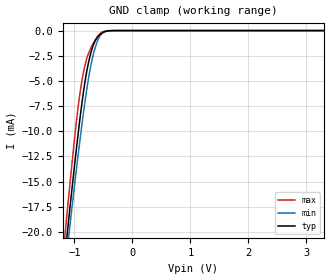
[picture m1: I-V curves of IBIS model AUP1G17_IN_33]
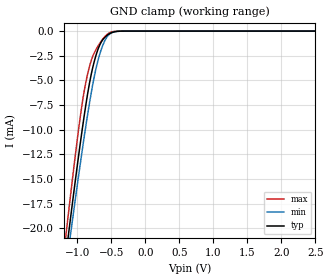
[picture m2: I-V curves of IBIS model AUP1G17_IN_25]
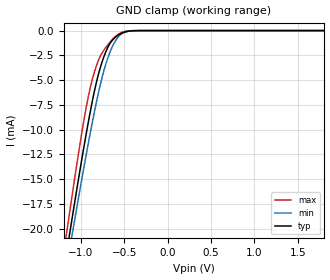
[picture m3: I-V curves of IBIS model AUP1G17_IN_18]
| TEXAS INSTRUMENTS INCORPORATED
| Standard Linear and Logic Group
| IBIS Model of SN74AUP1G17
| Low-Power Single Schmitt-Trigger Buffer
| This file contains package information for the following:
|  SOT 5-pin (DCK) package as [Component] AUP1G17_DCK
|  SOT 5-pin (DBV) package as [Component] AUP1G17_DBV
|  NanoStar WCSP 5-pin (YEP) package as [Component] AUP1G17_YEP
|  NanoFree WCSP 5-pin (YZP) package as [Component] AUP1G17_YZP
|  XSON 5-pin (DPW) package as [Component] AUP1G17_DPW
| This device can be powered at the following Vccs:
|  3.3 volt Vcc
|  2.5 volt Vcc
|  1.8 volt Vcc
|  1.5 volt Vcc
|  1.2 volt Vcc
|  0.8 volt Vcc
| This file provides unique models under the [Model Selector] for each Vcc.
| For operation at a specific Vcc, select the appropriate model after each
| [Model Selector] keyword.
[IBIS Ver]   3.2
[Comment char]  |_char
[File Name]   sn74aup1g17.ibs
[File Rev]   1.3 | a_die
[Date]   09/19/2017
[Source]   Data created from TI-SPICE simulations.
   Texas Instruments Incorporated.
   Analog-eLab, HPA
   12500 TI Blvd
   Dallas, TX -75243
   For Support e-mail: odt-pfmodeling@list.ti.com
[Notes]   The following is an IBIS list for the AUP1G17.
   - FILE REV HISTORY
   - 1.1 Release IBIS file on 04/02/04
   - 1.2 YEP and YZP packages released on 10/02/04
   - 1.3 DPW package released on 9/17/2017
   - Power clamp data deleted as there is no power-clamp diode.
   - Non-monotonic data in pullup data due to resistor at output
[Disclaimer]  This model is designed as an aid for customers of Texas Instruments
 TI and its licensors and suppliers make no warranties, either expressed
 or implied, with respect to this  model, including the warranties of
 merchantability or fitness for a particular purpose.
 The model is provided solely on an "as is" basis. The entire risk as to
 its quality and performance is with the customer.
[Copyright] (C)Copyright 2017 Texas Instruments Incorporated.
   All rights reserved.
| Component AUP1G17_DCK 5-pin SOT
[Component]   AUP1G17_DCK
[Manufacturer]   Texas Instruments, Inc.
[Package]
|   typ   min   max
R_pkg   2.000e-02   1.700e-02   2.500e-02
L_pkg   9.980e-10   8.810e-10   1.069e-09
C_pkg   1.460e-13   1.180e-13   2.050e-13
[Pin]   signal_name   model_name   R_pin   L_pin   C_pin
1   NC   NC   1.900e-02   1.069e-09   1.620e-13
2   A   AUP1G17_IN   1.800e-02   8.810e-10   1.210e-13
3   GND   GND   1.700e-02   1.031e-09   2.050e-13
4   Y   AUP1G17_OUT   2.000e-02   9.600e-10   1.240e-13
5   VCC   POWER   2.500e-02   1.049e-09   1.180e-13
| Component AUP1G17_DBV 5-pin SOT
[Component]   AUP1G17_DBV
[Manufacturer]   Texas Instruments, Inc.
[Package]
|   typ   min   max
R_pkg   2.500e-02   2.100e-02   2.900e-02
L_pkg   1.529e-09   1.312e-09   1.906e-09
C_pkg   1.560e-13   1.100e-13   2.400e-13
[Pin]   signal_name   model_name   R_pin   L_pin   C_pin
1   NC   NC   2.100e-02   1.511e-09   1.440e-13
2   A   AUP1G17_IN   2.300e-02   1.312e-09   1.380e-13
3   GND   GND   2.900e-02   1.906e-09   2.400e-13
4   Y   AUP1G17_OUT   2.600e-02   1.541e-09   1.500e-13
5   VCC   POWER   2.500e-02   1.374e-09   1.100e-13
| Component AUP1G17_YEP 5-pin NanoStar WCSP
[Component]   AUP1G17_YEP
[Manufacturer]   Texas Instruments, Inc.
[Package]
|   typ   min   max
R_pkg   0.001   0.001   0.001
L_pkg   0.021nH   0.021nH   0.021nH
C_pkg   0.046pF   0.045pF   0.047pF
[Pin]   signal_name   model_name   R_pin   L_pin   C_pin
1   DNU   NC   0.001   0.021nH   0.046pF
2   B   AUP1G17_IN   0.001   0.021nH   0.047pF
3   GND   GND   0.001   0.021nH   0.046pF
4   Y   AUP1G17_OUT   0.001   0.021nH   0.045pF
5   VCC   POWER   0.001   0.021nH   0.045pF
| Component AUP1G17_YZP 5-pin NanoStar WCSP
[Component]   AUP1G17_YZP
[Manufacturer]   Texas Instruments, Inc.
[Package]
|   typ   min   max
R_pkg   0.001   0.001   0.001
L_pkg   0.021nH   0.021nH   0.021nH
C_pkg   0.046pF   0.045pF   0.047pF
[Pin]   signal_name   model_name   R_pin   L_pin   C_pin
1   DNU   NC   0.001   0.021nH   0.046pF
2   B   AUP1G17_IN   0.001   0.021nH   0.047pF
3   GND   GND   0.001   0.021nH   0.046pF
4   Y   AUP1G17_OUT   0.001   0.021nH   0.045pF
5   VCC   POWER   0.001   0.021nH   0.045pF
| Component LVC1G38D_DPW 5-pin X2SON
[Component]   LVC1G38D_DPW
[Manufacturer]   Texas Instruments, Inc.
[Package]
|   typ   min   max
R_pkg   0.0364   0.0010   0.0518
L_pkg   0.2978n   0.0346n   0.4435n
C_pkg   0.0978p   0.0741p   0.1133p
[Pin]   signal_name   model_name   R_pin   L_pin   C_pin
1   D   LVC1G38D_IN   0.04116   0.30011n   0.10160p
2   CLK   LVC1G38D_IN   0.05181   0.44351n   0.11332p
3   GND   GND   0.00103   0.03456n   0.07412p
4   Q   LVC1G38D_OUT   0.04142   0.34311n   0.10148p
5   VCC   POWER   0.04662   0.36767n   0.09844p
| Model AUP1G17_IN
[Model Selector]   AUP1G17_IN
AUP1G17_IN_33   3.3 volt Vcc
AUP1G17_IN_25   2.5 volt Vcc
AUP1G17_IN_18   1.8 volt Vcc
AUP1G17_IN_15   1.5 volt Vcc
AUP1G17_IN_12   1.2 volt Vcc
AUP1G17_IN_08   0.8 volt Vcc
| Model AUP1G17_OUT
[Model Selector]   AUP1G17_OUT
AUP1G17_OUT_33   3.3 volt Vcc
AUP1G17_OUT_25   2.5 volt Vcc
AUP1G17_OUT_18   1.8 volt Vcc
AUP1G17_OUT_15   1.5 volt Vcc
AUP1G17_OUT_12   1.2 volt Vcc
AUP1G17_OUT_08   0.8 volt Vcc
| Models and submodels in the file (12): AUP1G17_IN_33 (Input), AUP1G17_IN_25 (Input), AUP1G17_IN_18 (Input), AUP1G17_IN_15 (Input), AUP1G17_IN_12 (Input), AUP1G17_IN_08 (Input), AUP1G17_OUT_33 (Output), AUP1G17_OUT_25 (Output), AUP1G17_OUT_18 (Output), AUP1G17_OUT_15 (Output), AUP1G17_OUT_12 (Output), AUP1G17_OUT_08 (Output)
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[Model]   AUP1G17_IN_33
Model_type  Input
Vinl=0.9
Vinh=2.1
| variable   typ   min   max
C_comp   1.44pF   1.17pF   1.80pF
[Temperature Range]   40   100   -40
| Ambient temperature   25   85   -40
[Voltage range]   3.3   3   3.6
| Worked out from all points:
|   GND clamp passes 1 mA (typ) near -0.64 V on its own axis
[GND Clamp]
| AUP1G17_IN_33
|   Voltage   I(typ)   I(min)   I(max)
-3.6V     -171.6mA   -163.5mA   -181.1mA
-1.16V    -22.22mA   -23.69mA   -20.18mA
-1.11V    -19.45mA   -21.09mA   -17.19mA
-1.085V   -18.08mA   -19.81mA   -15.71mA
-940mV    -10.5mA    -12.6mA    -7.822mA
-890mV    -8.117mA   -10.26mA   -5.698mA
-835mV    -5.768mA   -7.825mA   -3.925mA
-755mV    -3.153mA   -4.717mA   -2.255mA
-675mV    -1.463mA   -2.419mA   -1.277mA
-595mV    -617.7uA   -945.8uA   -546.7uA
-515mV    -215.4uA   -248.8uA   -134.4uA
3.3V      132.2pA    540.4pA    36.28pA
[Model]   AUP1G17_IN_25
Model_type  Input
Vinl=0.7
Vinh=1.6
| variable   typ   min   max
C_comp   1.47pF   1.22pF   1.80pF
[Temperature Range]   40   100   -40
| Ambient temperature   25   85   -40
[Voltage range]   2.5   2.3   2.7
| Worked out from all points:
|   GND clamp passes 1 mA (typ) near -0.64 V on its own axis
[GND Clamp]
| AUP1G17_IN_25
|   Voltage   I(typ)   I(min)   I(max)
-3.6V     -171.6mA   -163.5mA   -181.1mA
-1.165V   -22.5mA    -23.95mA   -20.48mA
-1.115V   -19.72mA   -21.35mA   -17.49mA
-1.09V    -18.36mA   -20.06mA   -16.01mA
-945mV    -10.75mA   -12.84mA   -8.061mA
-890mV    -8.117mA   -10.26mA   -5.698mA
-835mV    -5.768mA   -7.825mA   -3.925mA
-760mV    -3.287mA   -4.89mA    -2.329mA
-675mV    -1.463mA   -2.419mA   -1.277mA
-595mV    -617.7uA   -945.8uA   -546.7uA
-520mV    -233.1uA   -272.6uA   -149.9uA
2.5V      104.3pA    491.9pA    26.71pA
[Model]   AUP1G17_IN_18
Model_type  Input
Vinl=0.6825
Vinh=1.0725
| variable   typ   min   max
C_comp   1.51pF   1.28pF   1.78pF
[Temperature Range]   40   100   -40
| Ambient temperature   25   85   -40
[Voltage range]   1.8   1.65   1.95
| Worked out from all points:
|   GND clamp passes 1 mA (typ) near -0.64 V on its own axis
[GND Clamp]
| AUP1G17_IN_18
|   Voltage   I(typ)   I(min)   I(max)
-3.6V     -171.6mA   -163.5mA   -181.1mA
-1.16V    -22.22mA   -23.69mA   -20.18mA
-1.135V   -20.83mA   -22.39mA   -18.68mA
-1.11V    -19.45mA   -21.09mA   -17.19mA
-1.09V    -18.36mA   -20.06mA   -16.01mA
-960mV    -11.5mA    -13.57mA   -8.799mA
-850mV    -6.372mA   -8.471mA   -4.359mA
-780mV    -3.86mA    -5.615mA   -2.659mA
-710mV    -2.096mA   -3.313mA   -1.67mA
-625mV    -855.5uA   -1.409mA   -788.9uA
-540mV    -313.2uA   -390uA     -224.9uA
1.8V      83.14pA    451.3pA    18.98pA
